[IBIS Ver]   3.2
[File name]   chevelon_rev1p3.ibs
[File Rev]   1.2
[Date]   04/25/2006
[Source]   File originated at Intel Corporation.
[Notes]
Notes:
Created: 04/25/06
1) In order to properly use the PCIE models some
special handling is required.
Two driver models, a MAIN and EMPH must be placed in parallel.  Then the
main model is driven with the data pattern to be simulated, and the EMPH
model is driven with the main data pattern delayed by one bit time and
inverted.
MAIN = D[n]
EMPH = !D[n-1]
This equalization scheme has the effect of providing an enhanced signal
swing (where the main and both emphasis stages are all driving in the same
direction) at a logical bit transition.  For a run length of two or more the
first emphasis stages reverses and opposes the main drive causing a reduced
drive.
2) Rev 1.3 has the following modifications w.r.t Rev 1.2
DDR2 models based on B0 netlist
PCIE models based on B0 netlist
Package information extracted from sunrise lake pkg.
3) Signals with 'nc' for the model name are not necessarily no-connects. The
pins simply don't have a model in this IBIS file. Refer to the product
specification for proper usage of these pins.
4) Use the following buffer Strengths for the following interfaces:
DDR2:
srl_ddr_o_17_9   DDR2 20 Ohm buffer output only
srl_ddr_o_50   DDR2 50 Ohm buffer output only
srl_ddr_io_50   DDR2 50 Ohm buffer IO
srl_ddr_odt150   DDR2 ODT 150 Ohm
srl_ddr_odt75   DDR2 ODT 75 Ohm
PCIX:
pcix_m1_PL_22   For Mode 1
PCIE:
PCIE_MAIN_TX   pre-emphasis main buffer along with de-emphasis buffer,
PCIE_DEE_TX   pre-emphasis buffer
PCIE_CAP_TX   differential capacitance between both legs of the differential
   output driver
note: The PCIE_CAP_TX model is necessary to ensure accuracy.
   Use per following guideline:
   TYP corner simulation = 650fF model
   SLOW corner simulation = 900fF model
   FAST corner simulation = 500fF model
5) Running the ibis golden checker version 3.2 produces 63 Warnings which
have all been verified to be ok
6) In addition to the Package section having parasitics 3 clock input signals
also have parasitics below. These have exclusively been put in below because the
clock routes were very small and the parasitics were less than what is specified
in the package section
[Disclaimer]   This information is for modeling purposes only and is not
   guaranteed.
[Copyright]   Copyright 2006, Intel Corporation, All Rights Reserved.
[Component]   SunriseLake
[Manufacturer]  Intel Corporation
[Package]
|   typ   min   max
| Zero out the package default params if the package is modeled externally.
R_pkg   0.502Ohm   0.202Ohm   0.821Ohm
L_pkg   5.27nH   1.875nH   8.570nH
C_pkg   1.519pF   0.981pF   2.03pF
[Pin]   signal_name   model_name   R_pin   L_pin   C_pin
A37   0   nc
A36   0   nc
A35   vss   gnd
A34   nc   nc
A33   nc   nc
A32   nc   nc
A31   nc   nc
A30   nc   nc
A29   nc   nc
A28   nc   nc
A27   nc   nc
A26   nc   nc
A25   nc   nc
A24   vss   gnd
A23   nc   nc
A22   nc   nc
A21   vss   gnd
A20   nc   nc
A19   nc   nc
A18   vss   gnd
A17   nc   nc
A16   nc   nc
A15   vss   gnd
A14   nc   nc
A13   nc   nc
A12   vss   gnd
A11   gpio[1]   gpio_buf
A10   gpio[0]   gpio_buf
A9   xint#[1]   gpio_buf
A8   xint#[2]   gpio_buf
A7   hs_enum#   gpio_buf
A6   u0_rts#   gpio_buf
A5   u0_cts#   gpio_buf
A4   u1_cts#   gpio_buf
A3   vss   gnd
A2   0   nc
A1   0   nc
B37   0   nc
B36   vss   gnd
B35   nc   nc
B34   nc   nc
B33   nc   nc
B32   nc   nc
B31   nc   nc
B30   vss   gnd
B29   nc   nc
B28   nc   nc
B27   vss   gnd
B26   nc   nc
B25   nc   nc
B24   vss   gnd
B23   nc   nc
B22   nc   nc
B21   vss   gnd
B20   nc   nc
B19   nc   nc
B18   vss   gnd
B17   nc   nc
B16   nc   nc
B15   vss   gnd
B14   nc   nc
B13   nc   nc
B12   vss   gnd
B11   gpio[3]   gpio_buf
B10   vss   gnd
B9   xint#[3]   gpio_buf
B8   xint#[0]   gpio_buf
B7   vss   gnd
B6   u0_rxd   gpio_buf
B5   u0_txd   gpio_buf
B4   u1_txd   gpio_buf
B3   p_clko[3]   pcix_o
B2   vss   gnd
B1   0   nc
C37   vss   gnd
C36   dq[59]   ddr2_io_select
C35   dq[51]   ddr2_io_select
C34   vss   gnd
C33   ma[14]   ddr2_o_select
C32   nc   nc
C31   nc   nc
C30   nc   nc
C29   nc   nc
C28   nc   nc
C27   nc   nc
C26   nc   nc
C25   nc   nc
C24   vss   gnd
C23   nc   nc
C22   nc   nc
C21   vss   gnd
C20   nc   nc
C19   nc   nc
C18   vss   gnd
C17   nc   nc
C16   nc   nc
C15   vss   gnd
C14   nc   nc
C13   nc   nc
C12   vss   gnd
C11   gpio[7]   gpio_buf
C10   gpio[2]   gpio_buf
C9   xint#[5]   gpio_buf
C8   xint#[6]   gpio_buf
C7   hpi#   gpio_buf
C6   hs_lstat   gpio_buf
C5   u1_rxd   gpio_buf
C4   u1_rts#   gpio_buf
C3   p_clko[2]   pcix_o
C2   p_clko[0]   pcix_o
C1   vss   gnd
D37   dq[63]   ddr2_io_select
D36   dq[58]   ddr2_io_select
D35   dq[50]   ddr2_io_select
D34   dq[55]   ddr2_io_select
D33   nc   nc
D32   nc   nc
D31   nc   nc
D30   vss   gnd
D29   nc   nc
D28   nc   nc
D27   vss   gnd
D26   nc   nc
D25   nc   nc
D24   vss   gnd
D23   nc   nc
D22   nc   nc
D21   vss   gnd
D20   nc   nc
D19   nc   nc
D18   vss   gnd
D17   nc   nc
D16   nc   nc
D15   vss   gnd
D14   nc   nc
D13   nc   nc
D12   vss   gnd
D11   gpio[5]   gpio_buf
D10   vss   gnd
D9   xint#[4]   gpio_buf
D8   nmi0#   gpio_buf
D7   vss   gnd
D6   hs_freq[1]   gpio_buf
D5   nc   nc
D4   vss   gnd
D3   p_cal[2]   nc
D2   p_clkout   pcix_o
D1   p_clkin   gpio_i_buf   1.017   10.63n   2.26p
E37   dqs[7]   ddr2_io_select
E36   dq[62]   ddr2_io_select
E35   dqs[6]   ddr2_io_select
E34   dq[54]   ddr2_io_select
E33   vss   gnd
E32   nc   nc
E31   nc   nc
E30   nc   nc
E29   nc   nc
E28   nc   nc
E27   nc   nc
E26   nc   nc
E25   nc   nc
E24   vcc1p2   power
E23   vcc1p2   power
E22   vcc1p2   power
E21   nc   nc
E20   nc   nc
E19   vcc1p8   power
E18   vcc1p8   power
E17   vcc1p2   power
E16   nc   nc
E15   nc   nc
E14   vss   gnd
E13   vcc1p2   power
E12   vss   gnd
E11   gpio[6]   gpio_buf
E10   gpio[4]   gpio_buf
E9   xint#[7]   gpio_buf
E8   hs_led_out   gpio_buf
E7   nmi1#   gpio_buf
E6   hs_freq[0]   gpio_buf
E5   vcc3p3   power
E4   warm_rst#   gpio_i_buf
E3   nc   nc
E2   vss   gnd
E1   p_clko[1]   pcix_o
F37   dqs#[7]   ddr2_io_select
F36   vss   gnd
F35   dqs#[6]   ddr2_io_select
F34   vss   gnd
F33   odt[1]   ddr2_o_select
F32   vcc3p3   power
F31   nc   nc
F30   nc   nc
F29   nc   nc
F28   nc   nc
F27   nc   nc
F26   nc   nc
F25   nc   nc
F24   vcc1p2   power
F23   vcc1p2   power
F22   vcc1p2   power
F21   nc   nc
F20   nc   nc
F19   vcc1p8   power
F18   vcc1p8   power
F17   vss   gnd
F16   nc   nc
F15   nc   nc
F14   vcc1p2   power
F13   vss   gnd
F12   vcc1p2   power
F11   vcc3p3   power
F10   vcc3p3   power
F9   vcc3p3   power
F8   vcc3p3   power
F7   vcc3p3   power
F6   vcc3p3   power
F5   p_cal[0]   nc
F4   p_bmi   pcix_o
F3   p_cal[1]   nc
F2   p_rst#   gpio_i_buf
F1   p_rstout#   pcix_o
G37   dq[57]   ddr2_io_select
G36   dm[7]   ddr2_io_select
G35   dm[6]   ddr2_io_select
G34   dq[49]   ddr2_io_select
G33   cs#[1]   ddr2_o_select
G32   vcc3p3   power
G31   vcc3p3   power
G30   vcc3p3   power
G29   vcc3p3   power
G28   vcc3p3   power
G27   vcc3p3   power
G26   vcc3p3   power
G25   vcc3p3   power
G24   vcc1p2   power
G23   vcc1p2   power
G22   vcc1p2   power
G21   nc   nc
G20   nc   nc
G19   vcc1p8   power
G18   vcc1p8   power
G17   vss   gnd
G16   nc   nc
G15   nc   nc
G14   vss   gnd
G13   vcc1p2   power
G12   vcc1p2   power
G11   vss   gnd
G10   vcc1p2   power
G9   vss   gnd
G8   vcc1p2   power
G7   vss   gnd
G6   vcc3p3   power
G5   p_gnt#[3]   gpio_buf
G4   vss   gnd
G3   p_req#[2]   gpio_i_buf
G2   vss   gnd
G1   nc   nc
H37   dq[56]   ddr2_io_select
H36   dq[61]   ddr2_io_select
H35   dq[53]   ddr2_io_select
H34   dq[48]   ddr2_io_select
H33   ma[13]   ddr2_o_select
H32   vcc1p8   power
H31   vcc1p2x   power
H30   vss   gnd
H29   vcc1p2x   power
H28   vss   gnd
H27   vcc1p2x   power
H26   vss   gnd
H25   vcc1p2x   power
H24   vss   gnd
H23   vcc1p2   power
H22   vss   gnd
H21   vss   gnd
H20   vss   gnd
H19   vcc1p2   power
H18   vss   gnd
H17   vcc1p2   power
H16   vss   gnd
H15   vss   gnd
H14   vss   gnd
H13   vcc1p2   power
H12   vss   gnd
H11   vcc1p2   power
H10   vss   gnd
H9   vcc1p2   power
H8   vss   gnd
H7   vcc1p2   power
H6   vccvio   power
H5   vccvio   power
H4   p_req#[3]   gpio_i_buf
H3   p_gnt#[2]   gpio_buf
H2   nc   nc
H1   p_req#[1]   gpio_i_buf
J37   dq[60]   ddr2_io_select
J36   vss   gnd
J35   dq[52]   ddr2_io_select
J34   vss   gnd
J33   odt[0]   ddr2_o_select
J32   vcc1p8   power
J31   vss   gnd
J30   vcc1p2x   power
J29   vss   gnd
J28   vcc1p2x   power
J27   vss   gnd
J26   vcc1p2x   power
J25   vss   gnd
J24   vcc1p2   power
J23   vss   gnd
J22   vcc1p2   power
J21   vss   gnd
J20   vcc1p2   power
J19   vss   gnd
J18   vcc1p2   power
J17   vss   gnd
J16   vss   gnd
J15   vcc1p2   power
J14   vcc1p2   power
J13   vss   gnd
J12   vcc1p2   power
J11   vss   gnd
J10   vcc1p2   power
J9   vss   gnd
J8   vcc1p2   power
J7   vss   gnd
J6   vcc3p3   power
J5   p_gnt#[0]   gpio_buf
J4   p_gnt#[1]   gpio_buf
J3   nc   nc
J2   nc   nc
J1   p_req#[0]   gpio_i_buf
K37   dq[43]   ddr2_io_select
K36   vss   gnd
K35   dq[35]   ddr2_io_select
K34   vss   gnd
K33   cas#   ddr2_o_select
K32   vcc1p8   power
K31   vcc1p2x   power
K30   vss   gnd
K29   vcc1p2x   power
K28   vss   gnd
K27   vcc1p2x   power
K26   vss   gnd
K25   vcc1p2x   power
K24   vss   gnd
K23   vcc1p2x   power
K22   vss   gnd
K21   vcc1p2   power
K20   vss   gnd
K19   vcc1p2   power
K18   vss   gnd
K17   vcc1p2   power
K16   vss   gnd
K15   vcc1p2   power
K14   vss   gnd
K13   vcc1p2   power
K12   vss   gnd
K11   vcc1p2   power
K10   vss   gnd
K9   vcc1p2   power
K8   vss   gnd
K7   vcc1p2   power
K6   vcc3p3   power
K5   p_ad[31]   pcix_io_select
K4   vss   gnd
K3   p_ad[27]   pcix_io_select
K2   vss   gnd
K1   p_ad[29]   pcix_io_select
L37   dq[47]   ddr2_io_select
L36   dq[42]   ddr2_io_select
L35   dq[34]   ddr2_io_select
L34   dq[39]   ddr2_io_select
L33   we#   ddr2_o_select
L32   vcc1p8   power
L31   vss   gnd
L30   vcc1p2x   power
L29   vss   gnd
L28   vcc1p2x   power
L27   vss   gnd
L26   vcc1p2x   power
L25   vss   gnd
L24   vcc1p2x   power
L23   vss   gnd
L22   vcc1p2x   power
L21   vss   gnd
L20   vcc1p2   power
L19   vss   gnd
L18   vcc1p2   power
L17   vss   gnd
L16   vcc1p2   power
L15   vss   gnd
L14   vcc1p2   power
L13   vss   gnd
L12   vcc1p2   power
L11   vss   gnd
L10   vcc1p2   power
L9   vss   gnd
L8   vcc1p2   power
L7   vss   gnd
L6   vccvio   power
L5   vccvio   power
L4   p_ad[30]   pcix_io_select
L3   p_ad[28]   pcix_io_select
L2   p_ad[25]   pcix_io_select
L1   p_cbe#[3]   pcix_io_select
M37   dqs[5]   ddr2_io_select
M36   dq[46]   ddr2_io_select
M35   dqs[4]   ddr2_io_select
M34   dq[38]   ddr2_io_select
M33   vss   gnd
M32   vcc1p8   power
M31   vcc1p2x   power
M30   vss   gnd
M29   vcc1p2x   power
M28   vss   gnd
M27   vcc1p2x   power
M26   vss   gnd
M25   vcc1p2x   power
M24   vss   gnd
M23   vcc1p2x   power
M22   vss   gnd
M21   vcc1p2   power
M20   vss   gnd
M19   vcc1p2   power
M18   vss   gnd
M17   vcc1p2   power
M16   vss   gnd
M15   vcc1p2   power
M14   vss   gnd
M13   vcc1p2   power
M12   vss   gnd
M11   vcc1p2   power
M10   vss   gnd
M9   vcc1p2   power
M8   vss   gnd
M7   vcc1p2   power
M6   vccvio   power
M5   p_ad[26]   pcix_io_select
M4   p_ad[24]   pcix_io_select
M3   p_ad[23]   pcix_io_select
M2   p_ad[21]   pcix_io_select
M1   p_ad[19]   pcix_io_select
N37   dqs#[5]   ddr2_io_select
N36   vss   gnd
N35   dqs#[4]   ddr2_io_select
N34   vss   gnd
N33   cs#[0]   ddr2_o_select
N32   vcc1p8   power
N31   vss   gnd
N30   vcc1p2x   power
N29   vss   gnd
N28   vcc1p2x   power
N27   vss   gnd
N26   vcc1p2x   power
N25   vss   gnd
N24   vcc1p2x   power
N23   vss   gnd
N22   vcc1p2x   power
N21   vss   gnd
N20   vcc1p2   power
N19   vss   gnd
N18   vcc1p2   power
N17   vss   gnd
N16   vcc1p2   power
N15   vss   gnd
N14   vcc1p2   power
N13   vss   gnd
N12   vcc1p2   power
N11   vsspllp   gnd
N10   vcc1p2   power
N9   vss   gnd
N8   vcc1p2   power
N7   vss   gnd
N6   vcc3p3   power
N5   p_idsel   pcix_io_select
N4   vss   gnd
N3   p_ad[22]   pcix_io_select
N2   vss   gnd
N1   p_ad[17]   pcix_io_select
P37   dq[41]   ddr2_io_select
P36   dm[5]   ddr2_io_select
P35   dm[4]   ddr2_io_select
P34   dq[33]   ddr2_io_select
P33   ras#   ddr2_o_select
P32   vcc1p8   power
P31   vcc1p2x   power
P30   vss   gnd
P29   vcc1p2x   power
P28   vss   gnd
P27   vcc1p2x   power
P26   vss   gnd
P25   vcc1p2x   power
P24   vss   gnd
P23   vcc1p2x   power
P22   vss   gnd
P21   vcc1p2   power
P20   vss   gnd
P19   vcc1p2   power
P18   vss   gnd
P17   vcc1p2   power
P16   vss   gnd
P15   vcc1p2   power
P14   vss   gnd
P13   vcc1p2   power
P12   vss   gnd
P11   vcc1p2pllp   power
P10   vss   gnd
P9   vcc1p2   power
P8   vss   gnd
P7   vcc1p2   power
P6   vccvio   power
P5   vccvio   power
P4   p_ad[20]   pcix_io_select
P3   p_ad[18]   pcix_io_select
P2   p_cbe#[2]   pcix_io_select
P1   p_irdy#   pcix_io_select
R37   dq[40]   ddr2_io_select
R36   dq[45]   ddr2_io_select
R35   dq[37]   ddr2_io_select
R34   dq[32]   ddr2_io_select
R33   ba[0]   ddr2_o_select
R32   vcc1p8   power
R31   vss   gnd
R30   vcc1p2x   power
R29   vss   gnd
R28   vcc1p2x   power
R27   vss   gnd
R26   vcc1p2x   power
R25   vss   gnd
R24   vcc1p2x   power
R23   vss   gnd
R22   vcc1p2x   power
R21   vss   gnd
R20   vcc1p2   power
R19   vss   gnd
R18   vcc1p2   power
R17   vss   gnd
R16   vcc1p2   power
R15   vss   gnd
R14   vcc1p2   power
R13   vss   gnd
R12   vcc1p2   power
R11   vss   gnd
R10   vcc1p2   power
R9   vss   gnd
R8   vcc1p2   power
R7   vss   gnd
R6   vcc3p3   power
R5   p_ad[16]   pcix_io_select
R4   p_frame#   pcix_io_select
R3   p_devsel#   pcix_io_select
R2   p_pcixcap   nc
R1   p_perr#   pcix_io_select
T37   dq[44]   ddr2_io_select
T36   vss   gnd
T35   dq[36]   ddr2_io_select
T34   vss   gnd
T33   ma[10]   ddr2_o_select
T32   vcc1p8   power
T31   vcc1p2x   power
T30   vss   gnd
T29   vcc1p2x   power
T28   vss   gnd
T27   vcc1p2x   power
T26   vss   gnd
T25   vcc1p2x   power
T24   vss   gnd
T23   vcc1p2x   power
T22   vss   gnd
T21   vcc1p2   power
T20   vss   gnd
T19   vcc1p2   power
T18   vss   gnd
T17   vcc1p2   power
T16   vss   gnd
T15   vcc1p2   power
T14   vss   gnd
T13   vcc1p2   power
T12   vss   gnd
T11   vcc1p2   power
T10   vss   gnd
T9   vcc1p2   power
T8   vss   gnd
T7   vcc1p2   power
T6   vcc3p3   power
T5   p_trdy#   pcix_io_select
T4   vss   gnd
T3   p_stop#   pcix_io_select
T2   vss   gnd
T1   p_serr#   pcix_io_select
U37   cb[2]   ddr2_io_select
U36   cb[3]   ddr2_io_select
U35   m_ck#[2]   ddr2_o_select
U34   m_ck[2]   ddr2_o_select
U33   ba[1]   ddr2_o_select
U32   vcc1p8   power
U31   vss   gnd
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[Diff Pin] inv_pin  vdiff  tdelay_typ tdelay_min tdelay_max
AL35   AM35   0   0   0   0   | dqs[0]   dqs#[0]
AL37   AM37   0   0   0   0   | dqs[1]   dqs#[1]
AD35   AE35   0   0   0   0   | dqs[2]   dqs#[2]
AD37   AE37   0   0   0   0   | dqs[3]   dqs#[3]
M35   N35   0   0   0   0   | dqs[4]   dqs#[4]
M37   N37   0   0   0   0   | dqs[5]   dqs#[5]
E35   F35   0   0   0   0   | dqs[6]   dqs#[6]
E37   F37   0   0   0   0   | dqs[7]   dqs#[7]
W36   W37   0   0   0   0   | dqs[8]   dqs#[8]
W34   V34   0   0   0   0   | m_ck[0]   m_ck#[0]
AA35   AA34   0   0   0   0   | m_ck[1]   m_ck#[1]
U34   U35   0   0   0   0   | m_ck[2]   m_ck#[2]
AN20   AN19   0   0   0   0   | pe_calp   pe_caln
AU14   AT14   0   0   0   0   | perp[0]   pern[0]
AU15   AT15   0   0   0   0   | perp[1]   pern[1]
AU17   AT17   0   0   0   0   | perp[2]   pern[2]
AU18   AT18   0   0   0   0   | perp[3]   pern[3]
AU20   AT20   0   0   0   0   | perp[4]   pern[4]
AU21   AT21   0   0   0   0   | perp[5]   pern[5]
AU23   AT23   0   0   0   0   | perp[6]   pern[6]
AU24   AT24   0   0   0   0   | perp[7]   pern[7]
AR14   AP14   0   0   0   0   | petp[0]   petn[0]
AR15   AP15   0   0   0   0   | petp[1]   petn[1]
AR17   AP17   0   0   0   0   | petp[2]   petn[2]
AR18   AP18   0   0   0   0   | petp[3]   petn[3]
AR20   AP20   0   0   0   0   | petp[4]   petn[4]
AR21   AP21   0   0   0   0   | petp[5]   petn[5]
AR23   AP23   0   0   0   0   | petp[6]   petn[6]
AR24   AP24   0   0   0   0   | petp[7]   petn[7]
AK20   AK19   0   0   0   0   | refclkp   refclkn
[Series Pin Mapping] pin_2 model_name function_table_group
AR14   AP14  PCIE_CAP_TX
AR15   AP15  PCIE_CAP_TX
AR17   AP17  PCIE_CAP_TX
AR18   AP18  PCIE_CAP_TX
AR20   AP20  PCIE_CAP_TX
AR21   AP21  PCIE_CAP_TX
AR23   AP23  PCIE_CAP_TX
AR24   AP24  PCIE_CAP_TX
[Model Selector] ddr2_o_select
srl_ddr_o_17_9   output only 18 ohm buffer
srl_ddr_o_50   output only 50 Ohm buffer
[Model Selector] ddr2_io_select
srl_ddr_io_50   50 ohm IO ddr2 buffer
srl_ddr_odt150   Input Model for DDR II, with ODT 150 Ohm
srl_ddr_odt75   Input Model for DDR II, with ODT 75 Ohm
[Model Selector] pcix_io_select
pcix_m1_PL_18   I/O model for high voltage (3.3v) drive 18 ohm impedence
pcix_m1_PL_20   I/O model for high voltage (3.3v) drive 20 ohm impedence
pcix_m1_PL_22   I/O model for high voltage (3.3v) drive 22 ohm impedence
pcix_m1_PL_24   I/O model for high voltage (3.3v) drive 24 ohm impedence
pcix_m1_PL_26   I/O model for high voltage (3.3v) drive 26 ohm impedence
[Model Selector] pcie_o_select
PCIE_MAIN_TX   pre-emphasis main buffer
PCIE_DEE_TX   pre-emphasis boost buffer
[Model] PCIE_CAP_TX
Model_type Series
|   typ   min   max
C_comp   10.000fF   10.000fF   10.000fF
[Voltage Range]   1.800V   1.710V   1.890V
[Temperature Range]   60.0   105.0   0.0
| TYP MIN MAX
[C Series]   650fF   500fF   900fF
| Models and submodels in the file (18): gpio_buf (I/O), gpio_i_buf (Input), pcie_refclock (Input), PCIE_MAIN_TX (Output), PCIE_DEE_TX (Output), PCIE_CAP_TX (Series), pcie_rx (Input), pcix_o (Output), pcix_m1_PL_18 (I/O), pcix_m1_PL_20 (I/O), pcix_m1_PL_22 (I/O), pcix_m1_PL_24 (I/O), pcix_m1_PL_26 (I/O), srl_ddr_o_17_9 (Output), srl_ddr_o_50 (Output), srl_ddr_io_50 (I/O), srl_ddr_odt150 (Input), srl_ddr_odt75 (Input)
